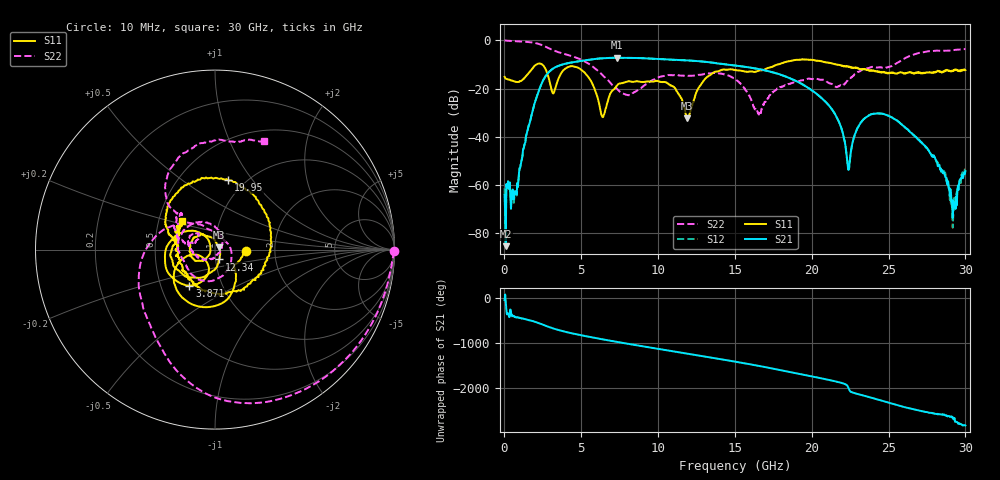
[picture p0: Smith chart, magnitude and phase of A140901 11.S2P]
!  2-Port S-parameters saved by WinCal
! VAR MeasName=S-Parameters (CALIBRATED_DATA) read from VNA (N5244A)
! VAR MeasDate=11/3/2014 9:27:37 AM
! VAR NAME=A140901 11
! VAR FILENAME=A140901 11.S2P
! VAR DATE=11/3/2014 9:27:37 AM
! VAR PHYS_PORTS=1,2
# Hz S RI R 50
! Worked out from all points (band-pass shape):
!   801 points, 10 MHz to 30 GHz, reference 50 ohm
!   highest |S21| = -7.22 dB at 7.32 GHz (marker M1); lowest = -85.5 dB at 84.97 MHz (marker M2)
!   |S21| within 3 dB of the highest: 3.67 GHz to 14.7 GHz (11.03 GHz wide, 120 % of centre)
!   lowest |S11| = -32.4 dB at 11.89 GHz (marker M3), VSWR 1.05, Z = 52.1 + j1.29 ohm
!   |S11| at or under -10 dB: start of sweep to 2.081 GHz; 2.451 GHz to 17.77 GHz (15.32 GHz wide, 152 % of centre); 21.65 GHz to end of sweep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
!   |S22| runs from -31.4 to 0.0 dB; largest |S21 - S12| = 0.0035
!   S11 on the Smith chart (normalised r, x): 10 MHz: 1.42, -0.01; 3.871 GHz: 0.70, -0.30; 12.34 GHz: 1.04, -0.12; 19.95 GHz: 0.84, +0.77; 30 GHz: 0.66, +0.22
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1e7  0.1749 -0.00502  0.00043 -0.000445  0.000635 0.000554  0.9972 -0.00914
8.4975e7  0.1595 -0.024  -4.82e-06 -5.28e-05  -2.5e-05 0.000123  0.9873 -0.0611
7.222625e8  0.11 -0.0842  0.000209 -0.000612  0.000385 -0.000562  0.8613 -0.4337
2.4092e9  -0.1845 -0.2657  -0.0922 0.0846  -0.0921 0.0845  -0.0429 -0.8059
3.15895e9  -0.0599 -0.0513  0.1918 0.1753  0.1911 0.175  -0.2972 -0.5522
3.871212e9  -0.1423 -0.2005  0.2883 -0.145  0.2878 -0.1447  -0.3907 -0.3533
5.033325e9  -0.2318 0.0643  -0.1532 -0.3441  -0.153 -0.3437  -0.3926 -0.0149
6.382875e9  -0.0256 0.000786  -0.3932 0.162  -0.3937 0.1611  -0.1223 0.1446
7.320062e9  -0.0955 -0.0632  -0.0739 0.4293  -0.0744 0.4286  -0.00914 0.0991
1.001916e10  -0.1377 0.0369  0.2322 -0.3401  0.2307 -0.3395  -0.00525 -0.1703
1.189354e10  0.0206 0.0124  -0.3615 -0.1294  -0.3615 -0.1289  -0.1635 -0.0825
1.234339e10  0.0235 -0.055  -0.3742 0.04  -0.3738 0.0394  -0.1763 -0.0574
1.5005e10  -0.2428 -0.00541  0.2818 0.1035  0.2823 0.1024  -0.0453 0.1501
1.654199e10  -0.2295 0.0547  0.0698 -0.2442  0.0694 -0.2445  0.025 -0.0192
1.995335e10  0.0734 0.3859  0.0548 0.0767  0.054 0.0768  -0.1467 0.058
2.002832e10  0.092 0.3844  0.059 0.0688  0.0586 0.0691  -0.1433 0.0622
2.239004e10  0.242 -0.1413  -0.00179 0.000977  -0.00167 0.00124  -0.1524 0.0322
2.332722e10  0.0436 -0.2512  0.0216 -0.00497  0.0216 -0.0049  -0.2234 0.1122
2.501416e10  -0.1621 -0.1261  -0.0268 -0.0013  -0.0269 -0.00127  -0.1966 0.2015
2.805065e10  -0.2051 0.0662  0.00142 -0.00306  0.00161 -0.00316  0.00285 0.6089
2.921276e10  -0.2057 0.1254  -0.000462 -6.39e-06  -5.32e-05 -0.000227  0.1602 0.6073
3e10  -0.1818 0.1574  0.00156 0.00111  0.00172 0.00117  0.2705 0.6027
